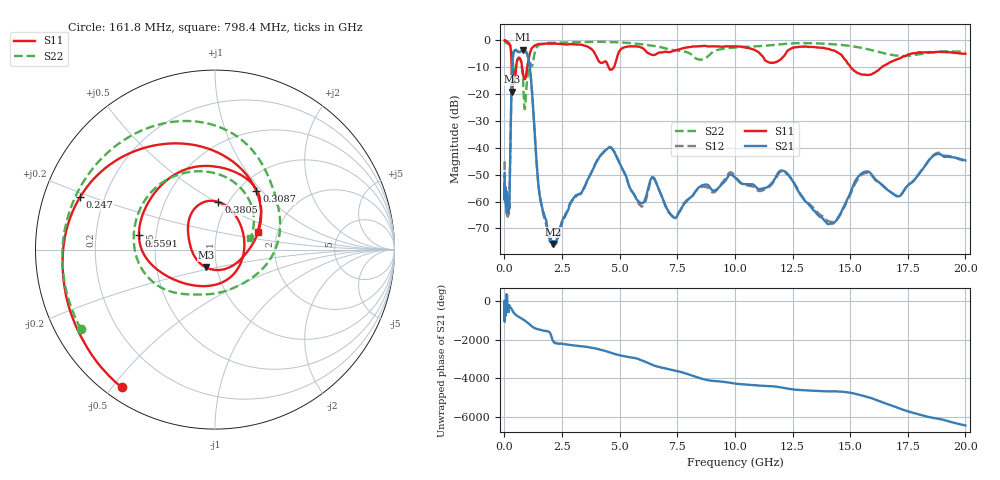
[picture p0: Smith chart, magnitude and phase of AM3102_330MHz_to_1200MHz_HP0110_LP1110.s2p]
! Date/Time: Tue, Sep 11, 2018 5:15 PM
! Network Analyzer: Agilent Technologies E8362B Rev: A.07.50.63
! Sweep from 0.010 to 20.000 GHz, 1601 Points, Sweep Type: LOG
! Power Supply: 4.949 V, 0.001 A
# Hz S DB R 50
!freq MagS11 AngS11 MagS21 AngS21 MagS12 AngS12 MagS22 AngS22
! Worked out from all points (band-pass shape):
!   1601 points, 10 MHz to 20 GHz, reference 50 ohm
!   highest |S21| = -3.41 dB at 821.5 MHz (marker M1); lowest = -75.8 dB at 2.104 GHz (marker M2)
!   |S21| within 3 dB of the highest: 366.7 MHz to 1.033 GHz (665.8 MHz wide, 95.2 % of centre)
!   lowest |S11| = -19.1 dB at 337.9 MHz (marker M3), VSWR 1.25, Z = 44.4 - j8.94 ohm
!   |S11| at or under -10 dB: 772 MHz to 989.2 MHz (217.3 MHz wide, 24.7 % of centre); 4.524 GHz to 4.749 GHz (224.7 MHz wide, 4.85 % of centre); 15.03 GHz to 16.37 GHz (1.34 GHz wide, 8.54 % of centre)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
!   |S22| runs from -25.6 to -0.3 dB; largest |S21 - S12| = 0.012
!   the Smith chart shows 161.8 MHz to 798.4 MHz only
!   S11 on the Smith chart (normalised r, x): 161.8 MHz: 0.05, -0.53; 247 MHz: 0.11, +0.19; 308.7 MHz: 1.21, +0.93; 380.5 MHz: 0.90, +0.51; 559.1 MHz: 0.40, +0.08; 798.4 MHz: 1.58, +0.34
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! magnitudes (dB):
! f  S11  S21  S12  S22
! 10 MHz  0.0  -49.4  -45.0  -0.3
! 35.55 MHz  0.0  -57.1  -58.7  -0.6
! 126.4 MHz  -0.4  -61.5  -62.5  -1.1
! 161.8 MHz  -0.7  -63.8  -63.4  -1.2
! 247 MHz  -1.9  -46.6  -46.7  -1.8
! 308.7 MHz  -8.0  -17.9  -17.9  -3.4
! 337.9 MHz  -19.1  -9.6  -9.6  -5.9
! 380.5 MHz  -11.5  -5.6  -5.7  -9.2
! 447.2 MHz  -15.2  -3.7  -3.7  -12.4
! 559.1 MHz  -7.3  -4.1  -4.1  -7.2
! 798.4 MHz  -11.8  -3.5  -3.5  -13.6
! 821.5 MHz  -13.0  -3.4  -3.5  -16.7
! 890.6 MHz  -14.4  -3.6  -3.7  -25.4
! 1.119 GHz  -4.4  -11.2  -11.3  -8.4
! 1.59 GHz  -1.3  -60.3  -60.4  -1.3
! 2.104 GHz  -1.2  -75.8  -76.4  -0.8
! 4.479 GHz  -9.0  -40.2  -40.1  -0.5
! 5.652 GHz  -2.2  -57.8  -57.7  -1.1
! 7.375 GHz  -3.8  -66.0  -65.9  -3.7
! 12.09 GHz  -6.1  -48.6  -48.9  -1.3
! 14.07 GHz  -3.2  -68.5  -67.3  -1.3
! 20 GHz  -4.9  -44.7  -45.2  -4.2
